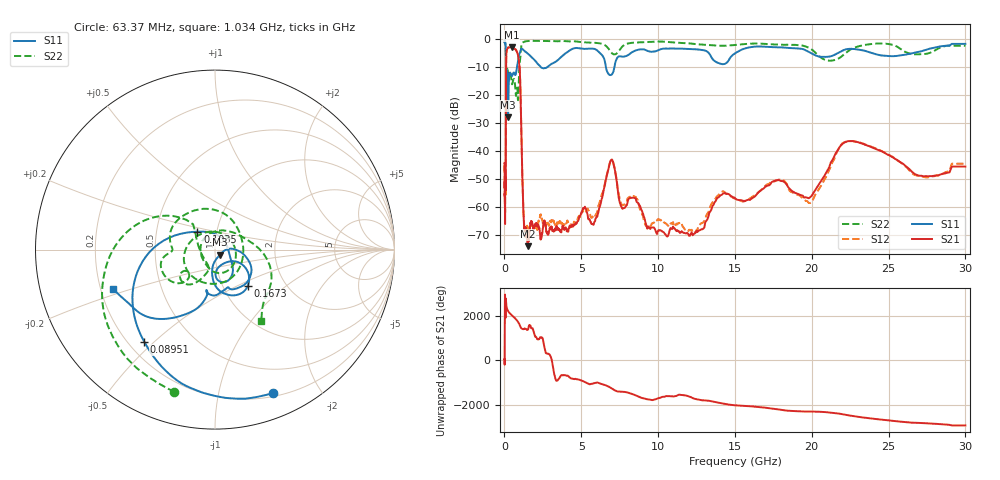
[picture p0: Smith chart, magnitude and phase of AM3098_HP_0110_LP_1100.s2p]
! Date/Time: Thu, Feb 28, 2019 8:38 AM
! Network Analyzer: Agilent Technologies E8364B Rev: A.07.50.67
! Sweep from 0.010 to 30.000 GHz, 1601 Points, Sweep Type: LOG
! Power Supply: 5.022 V, 0.001 A
# Hz S DB R 50
!freq MagS11 AngS11 MagS21 AngS21 MagS12 AngS12 MagS22 AngS22
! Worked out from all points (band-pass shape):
!   1601 points, 10 MHz to 30 GHz, reference 50 ohm
!   highest |S21| = -2.81 dB at 469 MHz (marker M1); lowest = -74.1 dB at 1.505 GHz (marker M2)
!   |S21| within 3 dB of the highest: 118.2 MHz to 888.8 MHz (770.7 MHz wide, 153 % of centre)
!   lowest |S11| = -27.9 dB at 237.5 MHz (marker M3), VSWR 1.08, Z = 52.9 - j2.97 ohm
!   |S11| at or under -10 dB: 99.92 MHz to 811.7 MHz (711.8 MHz wide, 156 % of centre); 2.376 GHz to 2.766 GHz (390.3 MHz wide, 15.2 % of centre); 6.609 GHz to 7.154 GHz (545.4 MHz wide, 7.93 % of centre)
!   |S22| runs from -22.2 to -0.5 dB; largest |S21 - S12| = 0.011
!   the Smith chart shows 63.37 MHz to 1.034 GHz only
!   S11 on the Smith chart (normalised r, x): 63.37 MHz: 0.23, -1.46; 89.51 MHz: 0.26, -0.47; 103.5 MHz: 0.81, +0.16; 167.3 MHz: 1.30, -0.57; 1.034 GHz: 0.25, -0.18
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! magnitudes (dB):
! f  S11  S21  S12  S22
! 10 MHz  -0.4  -44.2  -47.5  -0.6
! 38.04 MHz  -0.5  -60.3  -60.8  -0.9
! 63.37 MHz  -1.3  -52.0  -51.4  -1.7
! 89.51 MHz  -3.8  -41.3  -41.0  -4.1
! 103.5 MHz  -17.1  -13.2  -13.2  -20.8
! 144.7 MHz  -19.0  -3.8  -3.8  -14.0
! 167.3 MHz  -11.3  -3.5  -3.5  -10.6
! 237.5 MHz  -27.9  -2.9  -2.9  -12.2
! 469 MHz  -13.0  -2.8  -2.8  -15.3
! 550.5 MHz  -12.3  -3.1  -3.0  -14.9
! 885.5 MHz  -7.7  -5.7  -5.7  -21.7
! 1.034 GHz  -4.3  -16.7  -16.7  -6.5
! 1.244 GHz  -3.8  -63.3  -62.6  -0.9
! 1.505 GHz  -5.0  -74.1  -67.4  -0.6
! 2.084 GHz  -8.2  -66.9  -67.1  -0.5
! 5.812 GHz  -3.3  -66.3  -63.8  -1.2
! 6.924 GHz  -12.8  -43.3  -43.4  -4.4
! 7.926 GHz  -5.9  -59.6  -58.7  -1.6
! 12.13 GHz  -3.4  -69.6  -68.5  -1.5
! 19.9 GHz  -4.7  -56.5  -58.6  -3.3
! 22.56 GHz  -3.4  -36.4  -36.4  -3.5
! 30 GHz  -1.6  -45.6  -44.5  -2.3
